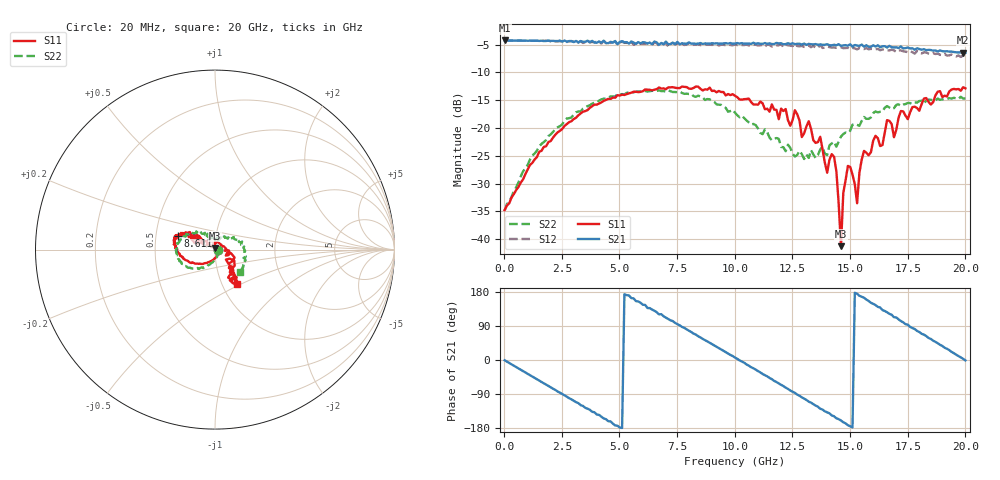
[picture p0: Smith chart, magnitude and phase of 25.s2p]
!Agilent Technologies,N5230A,US43500223,A.07.50.48
!Agilent N5230A: A.07.50.48
!Date: Tuesday, November 17, 2015 10:53:20
!Correction: S11(Full 2 Port(1,2))
!S21(Full 2 Port(1,2))
!S12(Full 2 Port(1,2))
!S22(Full 2 Port(1,2))
!S2P File: Measurements: S11, S21, S12, S22:
# Hz S  dB  R 50
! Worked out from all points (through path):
!   201 points, 20 MHz to 20 GHz, reference 50 ohm
!   highest |S21| = -4.24 dB at 20 MHz (marker M1); lowest = -6.5 dB at 19.9 GHz (marker M2)
!   group delay of S21, straight-line fit = 99.7 ps
!   lowest |S11| = -41.3 dB at 14.61 GHz (marker M3), VSWR 1.02, Z = 49.9 + j0.856 ohm
!   |S11| at or under -10 dB: start of sweep to end of sweep
!   |S22| runs from -34.9 to -13.2 dB; largest |S21 - S12| = 0.066
!   S11 on the Smith chart (normalised r, x): 20 MHz: 1.04, -0.00; 8.611 GHz: 0.65, +0.10; 20 GHz: 1.17, -0.48
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2e7  -34.77 -1.5  -4.24 -0.7  -4.23 -0.7  -34.93 0.9
1.9181e9  -22.54 -114.4  -4.28 -68.3  -4.28 -69.3  -21.46 -107.6
3.4166e9  -17.07 -147.9  -4.47 -121.2  -4.69 -123.2  -16.52 -134.9
5.1149e9  -14.00 -172.7  -4.35 -179.4  -4.47 177.7  -13.90 -158.2
6.7133e9  -12.70 172.7  -5.02 120.5  -5.16 118.7  -13.21 -178.4
8.6114e9  -13.24 159.9  -4.86 55.7  -5.08 52.9  -14.48 156.5
1.001e10  -14.20 153.3  -4.78 6.4  -4.93 3.3  -17.25 136.1
1.2008e10  -16.50 154.4  -4.74 -65.6  -4.83 -68.6  -23.42 116.6
1.34066e10  -22.20 141.2  -4.95 -116.6  -5.20 -120.4  -24.77 99.7
1.37063e10  -21.58 149.7  -4.93 -128.6  -5.04 -130.8  -23.86 82.3
1.4006e10  -28.05 143.1  -4.90 -138.2  -5.35 -141.0  -24.88 69.5
1.43057e10  -25.20 117.2  -5.01 -148.6  -5.49 -153.5  -22.49 65.1
1.46054e10  -41.28 96.4  -5.21 -159.7  -5.45 -164.7  -21.55 52.1
1.47053e10  -31.69 143.8  -5.12 -164.3  -5.62 -167.6  -21.08 55.8
1.49051e10  -26.83 73.4  -5.18 -172.2  -5.56 -175.8  -20.92 48.3
1.53047e10  -33.55 14.7  -5.15 174.6  -5.84 170.6  -19.43 39.1
1.56044e10  -24.13 4.1  -5.35 164.3  -5.78 159.4  -18.01 33.8
1.67033e10  -18.71 -35.7  -5.21 121.8  -6.03 118.8  -16.31 14.0
1.69031e10  -21.65 -42.5  -5.49 112.9  -6.01 109.0  -16.43 10.4
1.82018e10  -14.70 -52.8  -5.81 66.9  -6.37 64.1  -15.62 -16.2
1.99001e10  -12.66 -56.3  -6.45 3.2  -6.97 -0.7  -14.69 -40.4
2e10  -12.86 -57.8  -6.45 -1.0  -6.97 -5.6  -14.71 -42.0
